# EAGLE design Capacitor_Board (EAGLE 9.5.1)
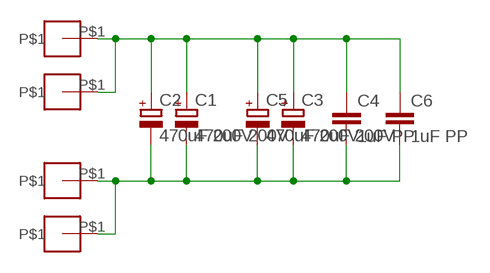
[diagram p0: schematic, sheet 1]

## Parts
C1  470uF 200V  CPOL-EUE10-25  [EB25D]
C2  470uF 200V  CPOL-EUE10-22.5  [EB22,5D]
C3  470uF 200V  CPOL-EUE10-22.5  [EB22,5D]
C4  1uF PP  C-EU102-064X133  [C102-064X133]
C5  470uF 200V  CPOL-EUE10-25  [EB25D]
C6  1uF PP  C-EU102-064X133  [C102-064X133]
U$1  BIG_PINHEADX1M4  [M4_PINHEAD]
U$2  BIG_PINHEADX1M4  [M4_PINHEAD]
U$3  BIG_PINHEADX1M4  [M4_PINHEAD]
U$4  BIG_PINHEADX1M4  [M4_PINHEAD]

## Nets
B+: C1.+ C2.+ C3.+ C4.1 C5.+ C6.1 U$1.P$1 U$3.P$1
B-: C1.- C2.- C3.- C4.2 C5.- C6.2 U$2.P$1 U$4.P$1

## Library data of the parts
C1-C3 C5 = resistor:CPOL-EU: POLARIZED CAPACITOR, European symbol
C4 C6 = resistor:C-EU: CAPACITOR, European symbol
U$1-U$4 = Ians parts:BIG_PINHEADX1

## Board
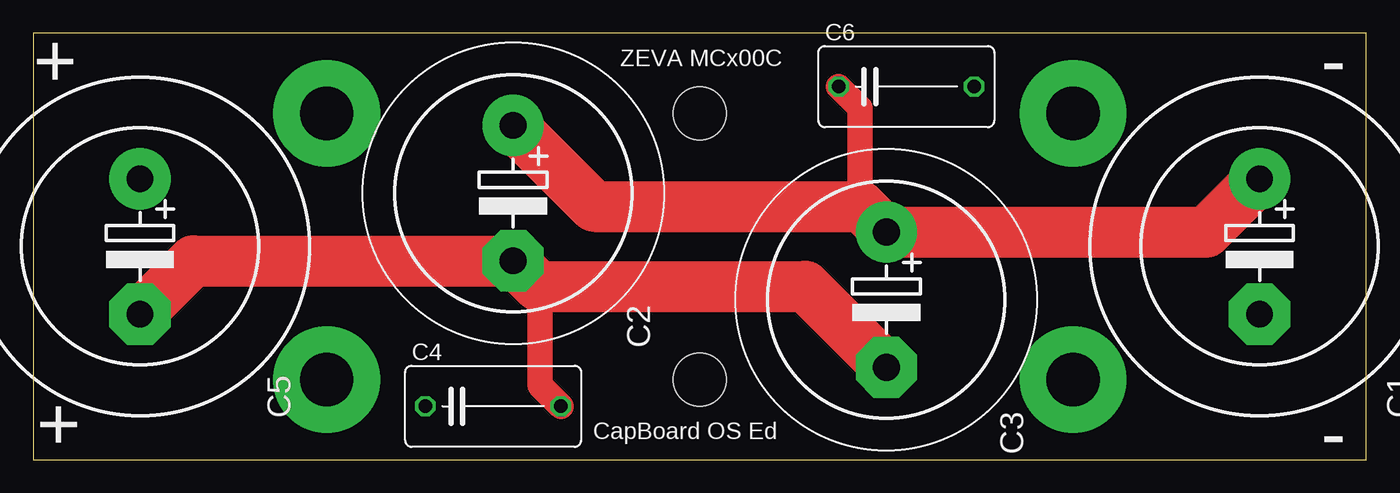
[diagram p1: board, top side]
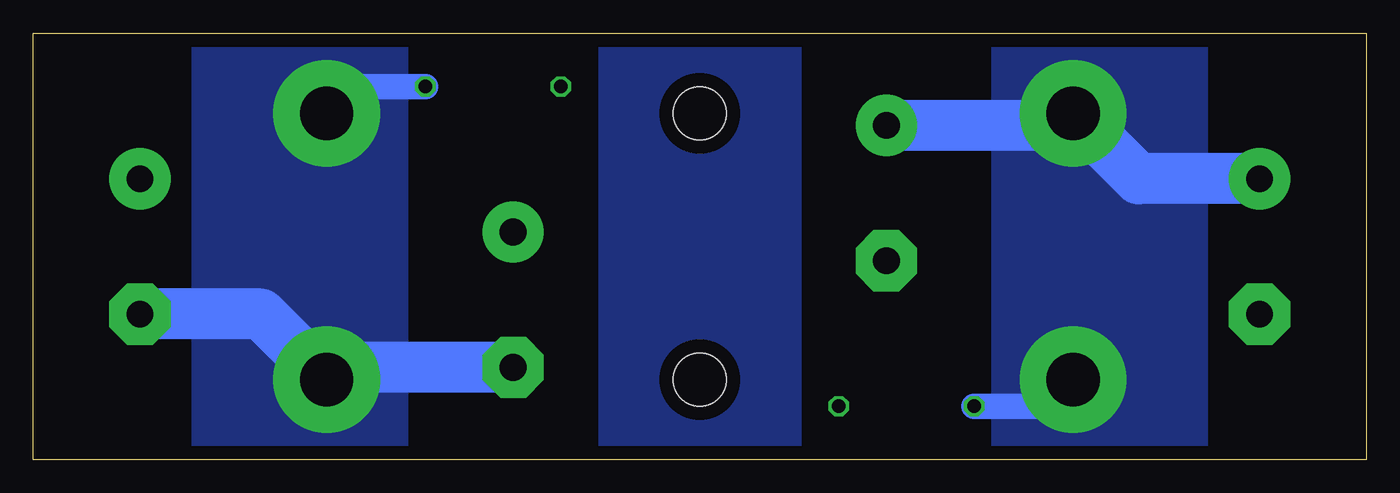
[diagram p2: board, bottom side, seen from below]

Size 100 x 32 mm. Coordinates in mm from the lower left corner, seen from the top.
Outline: 0,0 100,0 100,32 0,32 0,0
Copper layers (1*16): Top 0.035mm / dielectric 1.5mm / Bottom 0.035mm
Design rules "default": minimum track width 10mil, minimum drill 24mil, track to track 8mil, track to pad 8mil, pad to pad 8mil, via to via 8mil, smd to smd 8mil, copper to edge 40mil, drill to drill 8mil, minimum pad ring 10mil, minimum via ring 8mil, stop-mask expansion 4mil, vias tented up to drill 0mil, thermal gap 10mil
Holes 4 mm at 50,26 50,6

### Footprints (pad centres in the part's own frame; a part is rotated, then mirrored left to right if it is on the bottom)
EB25D = drill 2.007 pad 4.597: + -5.08,0 | drill 2.007 pad 4.597 octagon: - 5.08,0
EB22,5D = drill 2.007 pad 4.597: + -5.08,0 | drill 2.007 pad 4.597 octagon: - 5.08,0
C102-064X133 = drill 1.016 octagon: 1 -5.08,0; 2 5.08,0
M4_PINHEAD = drill 4 pad 8: P$1 0,0

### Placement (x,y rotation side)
C1  92,16 270 top
C2  36,20 270 top
C3  64,12 270 top
C4  34.5,4 0 top
C5  8,16 270 top
C6  65.5,28 0 top
U$1  22,6 0 top
U$2  78,26 0 top
U$3  22,26 0 top
U$4  78,6 0 top

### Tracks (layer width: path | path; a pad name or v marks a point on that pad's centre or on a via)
B+
  Top 1.93: C6.1 62,26.42 62,19
  Top 3.81: C1.+ 88,17.08 C3.+ 62.08,19 62,19 42.08,19 C2.+
  Bottom 1.93: U$1.P$1 24,4 C4.1
  Bottom 3.81: C5.+ 17.08,21.08 U$3.P$1 22.92,25.08 C2.+
  pour Bottom: 12,33 28,33 28,-1 12,-1
B-
  Top 1.93: C4.2 38,5.58 38,13
  Top 3.81: C5.- 12,14.92 C2.- 37.92,13 38,13 57.92,13 C3.-
  Bottom 1.93: U$2.P$1 76,28 C6.2
  Bottom 3.81: C3.- 77.08,6.92 U$4.P$1 82.92,10.92 C1.-
  pour Bottom: 72,33 88,33 88,-1 72,-1
DUMMY
  pour Bottom: 42.5,33 57.5,33 57.5,-1 42.5,-1

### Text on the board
tPlace: + | ZEVA MCx00C | - | CapBoard OS Ed | + | -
